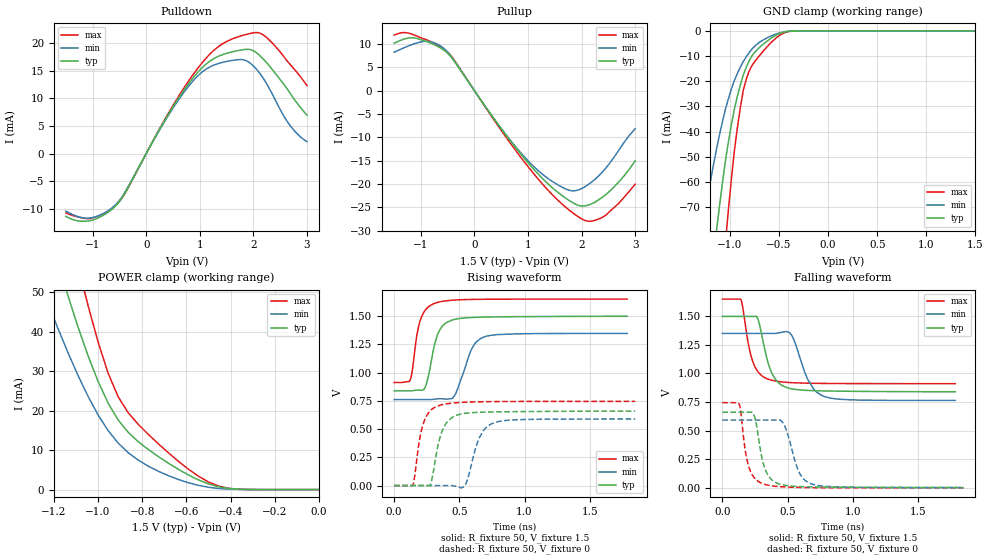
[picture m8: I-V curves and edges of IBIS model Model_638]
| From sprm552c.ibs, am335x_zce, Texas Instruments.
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| Model based on original model for BCSHTLTCSCDDVPBFZ_SSDHV
|   Sub model SR00_6MA_PADP_10PER_1P5
[model]   Model_638
|[Description]  [1.5V-3-STATE-NOTERM-SR00:6MA, IND, 10%]
|   Fastest slew rate (SR[1:0] = "00"), 1.33 * RExt = 0.750 * Iout
|   (I[2:0] = "001"), 6mA nominal with Rext = 50R,ODT off (ODT[1:0]
|   = "00") CMOS mode,Industrial temperature range (-40C to 125C,
|   25C nominal),10% power supply tolerance
|[Input Load]   NOTERM
|[Output Drive] SR00:6MA
|Voltage   1.5V
|Mode   3-STATE
Model_type   3-state
Polarity   Non-Inverting
Enable   Active-Low
Cref =  15pF
Rref =  100.0000M
Vref =  0V
Vmeas =  0.75
C_comp   1.865048p   1.676829p   1.989968p
[Temperature Range]   25   125   -40
[Voltage Range]   1.5   1.35   1.65
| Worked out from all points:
|   slope of the pulldown table from 0 to 0.225 V, typ, clamps not added: 56.6 ohm
|   slope of the pullup table from 0 to 0.225 V, typ, clamps not added: 60 ohm
|   GND clamp passes 1 mA (typ) near -0.49 V on its own axis
|   POWER clamp passes 1 mA (typ) near -0.47 V on its own axis
|   rising waveform, R_fixture 50, V_fixture 1.5: 20-80 % time 82.3ps typ, 111ps min, 69.4ps max; typ from 0.839 V to 1.5 V
|   rising waveform, R_fixture 50, V_fixture 0: 20-80 % time 83.8ps typ, 98.4ps min, 74.9ps max; typ from 0 V to 0.658 V
|   falling waveform, R_fixture 50, V_fixture 1.5: 20-80 % time 97.7ps typ, 122ps min, 83.3ps max; typ from 1.5 V to 0.841 V
|   falling waveform, R_fixture 50, V_fixture 0: 20-80 % time 73.9ps typ, 95.9ps min, 65.8ps max; typ from 0.661 V to 0.002 V
[POWER_clamp]
-1.5V     126mA      88.79mA    168.7mA
-1.242V   69.8mA     49.45mA    94.34mA
-1.136V   49.16mA    34.72mA    67.51mA
-1.061V   36.35mA    25.4mA     50.03mA
-1.045V   33.92mA    23.63mA    46.66mA
-954.5mV  21.93mA    14.95mA    29.5mA
-909.1mV  17.64mA    11.79mA    23.52mA
-863.6mV  14.51mA    9.351mA    19.47mA
-772.7mV  10.16mA    5.94mA     13.99mA
-590.9mV  3.705mA    1.741mA    5.166mA
-454.5mV  710.5uA    279.1uA    892.1uA
0V        1.424nA    14.34nA    3.127nA
[Pulldown]
-1.5V     -11.35mA   -10.4mA    -10.74mA
-1V       -12.02mA   -11.55mA   -11.65mA
-727.3mV  -10.71mA   -10.42mA   -10.5mA
-500mV    -8.674mA   -8.454mA   -8.641mA
272.7mV   4.789mA    4.647mA    4.892mA
681.8mV   11.16mA    10.78mA    11.53mA
1.045V    15.53mA    14.75mA    16.42mA
1.364V    17.65mA    16.32mA    19.44mA
1.818V    18.79mA    16.93mA    21.4mA
2.136V    17.56mA    14.29mA    21.7mA
2.636V    11.62mA    5.736mA    16.68mA
3V        6.943mA    2.158mA    12.3mA
[Pullup]
-1.5V     10.19mA    8.245mA    11.94mA
-1.182V   11.36mA    9.829mA    12.18mA
-954.5mV  10.77mA    10.55mA    11.16mA
-590.9mV  8.854mA    9.241mA    9.128mA
-409.1mV  6.831mA    6.942mA    7.07mA
909.1mV   -14.2mA    -13.89mA   -14.94mA
1.318V    -19.37mA   -18.35mA   -20.63mA
1.773V    -23.58mA   -21.37mA   -25.64mA
2.045V    -24.72mA   -20.72mA   -27.74mA
2.318V    -23.4mA    -18.26mA   -27.52mA
2.682V    -19.71mA   -12.98mA   -24.27mA
3V        -15.03mA   -8.169mA   -20.07mA
[GND_clamp]
-1.5V     -219.3mA   -131.6mA   -364.3mA
-1.288V   -134.4mA   -79.74mA   -225.6mA
-1.258V   -122.9mA   -72.77mA   -206.3mA
-1.136V   -79.27mA   -46.88mA   -132.4mA
-1.045V   -51.5mA    -31.06mA   -84.11mA
-1.015V   -44.02mA   -26.9mA    -70.91mA
-954.5mV  -31.01mA   -19.7mA    -47.55mA
-863.6mV  -17.48mA   -12.16mA   -23.55mA
-803mV    -11.81mA   -8.597mA   -15.85mA
-681.8mV  -5.986mA   -4.096mA   -9.026mA
-378.8mV  -126.2uA   -131.8uA   -179.7uA
1.5V      1.424nA    207.1nA    1.498nA
[Ramp]
dV/dt_f 0.40407685/98.562939p 0.36253871/0.12245143n 0.44853436/83.46658p
dV/dt_r  0.4039305/84.698658p 0.36650846/99.684603p 0.45218119/74.873543p
R_load = 50
[Rising Waveform]
R_fixture = 50
V_fixture = 1.5
V_fixture_min = 1.35
V_fixture_max = 1.65
0s        838.7mV    760.8mV    912.1mV
123.5ps   838.7mV    760.8mV    935.2mV
184.4ps   844.6mV    760.8mV    1.39V
227.6ps   851.1mV    760.8mV    1.533V
314ps     1.265V     765.4mV    1.614V
370.2ps   1.412V     767.9mV    1.63V
455.6ps   1.469V     782.7mV    1.641V
596.7ps   1.488V     1.214V     1.647V
691.9ps   1.491V     1.316V     1.649V
1.787ns   1.498V     1.347V     1.65V
[Rising Waveform]
R_fixture = 50
V_fixture = 0
V_fixture_min = 0
V_fixture_max = 0
0s        0V         0V         0V
142.7ps   0V         0V         0V
208.5ps   0V         0V         482.9mV
275.5ps   0V         0V         659.4mV
339ps     368.4mV    0V         706.3mV
400.7ps   554.6mV    0V         723.3mV
538.8ps   638.3mV    -7.584mV   737mV
651.1ps   648.4mV    416.7mV    741.1mV
757.1ps   651.6mV    551.3mV    743mV
1.848ns   658.4mV    589.1mV    744.9mV
[Falling Waveform]
R_fixture = 50
V_fixture = 1.5
V_fixture_min = 1.35
V_fixture_max = 1.65
0s        1.499V     1.351V     1.65V
140.5ps   1.499V     1.351V     1.65V
211.7ps   1.499V     1.351V     1.192V
264ps     1.499V     1.351V     1.03V
351.2ps   1.092V     1.351V     950.2mV
417.8ps   933.6mV    1.352V     931.9mV
514.4ps   870.3mV    1.359V     921.1mV
656.1ps   851.8mV    945.2mV    915.2mV
783.6ps   847.3mV    798.4mV    913.1mV
1.787ns   840.6mV    765mV      911.2mV
[Falling Waveform]
R_fixture = 50
V_fixture = 0
V_fixture_min = 0
V_fixture_max = 0
0s        660.8mV    593mV      744.6mV
127.7ps   660.8mV    593mV      735.9mV
183.7ps   660.8mV    593mV      274.6mV
238.8ps   646.6mV    593mV      97.2mV
316.9ps   201.3mV    593mV      33.67mV
371.3ps   78.3mV     593mV      18.97mV
458.2ps   27.35mV    578.6mV    9.137mV
593.5ps   11.23mV    125mV      3.804mV
694.5ps   8.139mV    30.28mV    2.141mV
1.848ns   2.308mV    3.353mV    0V
